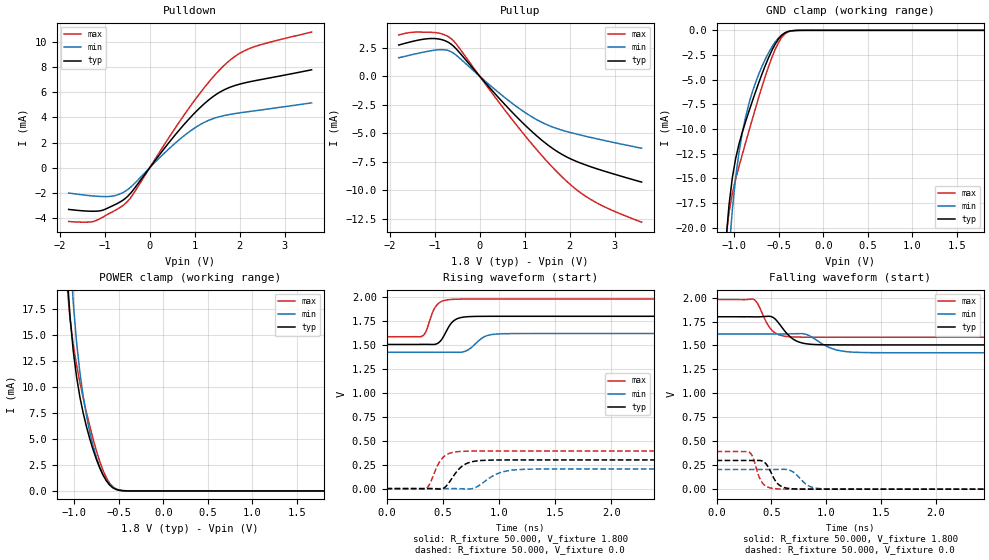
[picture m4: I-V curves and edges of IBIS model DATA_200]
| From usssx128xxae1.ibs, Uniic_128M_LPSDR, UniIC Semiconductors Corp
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|   Model DATA_200
[Model] DATA_200
Model_type I/O
Polarity   Inverting
Enable   Active-High
Vinl =  0.0V
Vinh =  1.800V
Vmeas =  0.900V
Vref =  0.900V
C_comp   1.060pF   1.050pF   1.070pF
[Model Spec]
Vinh   1.800V   1.400V   2.100V
Vinl   0.0V   -0.300V   0.400V
Vmeas   0.900V   0.810V   0.990V
Vref   0.900V   0.810V   0.990V
[Temperature Range]   25.000   0.125k   -40.000
[Voltage Range]   1.800V   1.620V   1.980V
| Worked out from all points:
|   slope of the pulldown table from 0 to 0.27 V, typ, clamps not added: 212 ohm
|   slope of the pullup table from 0 to 0.27 V, typ, clamps not added: 221 ohm
|   GND clamp passes 1 mA (typ) near -0.51 V on its own axis
|   POWER clamp passes 1 mA (typ) near -0.64 V on its own axis
|   rising waveform, R_fixture 50.000, V_fixture 1.800: 20-80 % time 91.8ps typ, 118ps min, 77.4ps max; typ from 1.51 V to 1.8 V
|   rising waveform, R_fixture 50.000, V_fixture 0.0: 20-80 % time 125ps typ, 171ps min, 97.4ps max; typ from 0 V to 0.3 V
|   falling waveform, R_fixture 50.000, V_fixture 1.800: 20-80 % time 139ps typ, 185ps min, 109ps max; typ from 1.8 V to 1.51 V
|   falling waveform, R_fixture 50.000, V_fixture 0.0: 20-80 % time 88.5ps typ, 114ps min, 72.7ps max; typ from 0.3 V to 0 V
[Pulldown]
|Voltage   I(typ)   I(min)   I(max)
-1.8V     -3.295mA   -1.994mA   -4.25mA
-1.195V   -3.435mA   -2.245mA   -4.185mA
-1.03V    -3.339mA   -2.275mA   -3.883mA
-810mV    -2.983mA   -2.23mA    -3.454mA
-480mV    -2.229mA   -1.703mA   -2.619mA
400mV     1.869mA    1.411mA    2.243mA
895mV     3.949mA    2.895mA    4.836mA
1.39V     5.592mA    3.872mA    7.11mA
1.83V     6.441mA    4.26mA     8.654mA
2.05V     6.676mA    4.38mA     9.168mA
2.325V    6.891mA    4.511mA    9.59mA
3.6V      7.767mA    5.147mA    10.75mA
[Pullup]
|Voltage   I(typ)   I(min)   I(max)
-1.8V     2.731mA    1.612mA    3.624mA
-1.46V    3.081mA    1.927mA    3.861mA
-1.075V   3.305mA    2.238mA    3.848mA
-855mV    3.219mA    2.33mA     3.728mA
-635mV    2.812mA    2.146mA    3.296mA
-470mV    2.17mA     1.67mA     2.561mA
905mV     -3.895mA   -2.906mA   -4.718mA
1.4V      -5.677mA   -4.087mA   -7.046mA
1.84V     -6.889mA   -4.75mA    -8.873mA
2.225V    -7.596mA   -5.151mA   -10.18mA
2.555V    -8.063mA   -5.453mA   -11.01mA
3.6V      -9.294mA   -6.325mA   -12.82mA
[GND_clamp]
|Voltage   I(typ)   I(min)   I(max)
-1.8V     -271.7mA   -304.3mA   -257.9mA
-1.097V   -21.71mA   -28.04mA   -21.32mA
-1.06V    -17.73mA   -22.52mA   -18.46mA
-1.023V   -14.97mA   -18.24mA   -16.55mA
-986mV    -13.03mA   -14.97mA   -15.09mA
-912mV    -10.37mA   -10.44mA   -12.62mA
-801mV    -7.262mA   -6.333mA   -9.099mA
-690mV    -4.437mA   -3.666mA   -5.721mA
-579mV    -2.043mA   -1.694mA   -2.765mA
-431mV    -248.4uA   -247.4uA   -345.1uA
-283mV    -5.293uA   -10.2uA    -5.65uA
1.8V      0A         0A         0A
[POWER_clamp]
|Voltage   I(typ)   I(min)   I(max)
-1.8V     340.2mA    394mA      317.1mA
-1.086V   21.52mA    29.62mA    20.16mA
-1.049V   16.79mA    23.07mA    16.54mA
-1.012V   13.42mA    18.08mA    14.02mA
-975mV    10.94mA    14.29mA    12.08mA
-938mV    9.034mA    11.39mA    10.43mA
-901mV    7.488mA    9.092mA    8.933mA
-827mV    5.01mA     5.66mA     6.217mA
-716mV    2.228mA    2.327mA    2.865mA
-568mV    301.3uA    355.6uA    397.2uA
-420mV    7.103uA    18.41uA    6.039uA
1.8V      0A         0A         0A
[Ramp]
| variable   typ   min   max
dV/dt_r   0.180/0.125n   0.123/0.171n   0.236/97.547p
dV/dt_f   0.176/0.139n   0.117/0.185n   0.236/0.110n
R_load = 50.000
[Rising Waveform]
R_fixture= 50.000
V_fixture= 1.800
V_fixture_min= 1.620
V_fixture_max= 1.980
|time   V(typ)   V(min)   V(max)
0s        1.506V     1.424V     1.586V
320ps     1.507V     1.424V     1.595V
353ps     1.507V     1.424V     1.647V
413ps     1.506V     1.424V     1.85V
443ps     1.511V     1.424V     1.912V
607ps     1.761V     1.424V     1.978V
713ps     1.795V     1.442V     1.98V
879ps     1.8V       1.592V     1.98V
1.031ns   1.8V       1.618V     1.98V
10ns      1.8V       1.62V      1.98V
[Rising Waveform]
R_fixture= 50.000
V_fixture= 0.0
V_fixture_min= 0.0
V_fixture_max= 0.0
|time   V(typ)   V(min)   V(max)
0s        16.25nV    102.8nV    27.47nV
352ps     578.9uV    32.05uV    -749.8uV
462ps     -4.438mV   4.627uV    259.9mV
502ps     991.9uV    179.1uV    325.3mV
580ps     104.6mV    506.8uV    375.5mV
706ps     259mV      -3.453mV   390.8mV
789ps     287.1mV    10.72mV    392.4mV
1.028ns   299.1mV    173.4mV    392.9mV
1.268ns   299.6mV    203.1mV    392.9mV
10ns      299.6mV    205.7mV    392.9mV
[Falling Waveform]
R_fixture= 50.000
V_fixture= 1.800
V_fixture_min= 1.620
V_fixture_max= 1.980
|time   V(typ)   V(min)   V(max)
0s        1.8V       1.62V      1.98V
337ps     1.799V     1.62V      1.982V
371ps     1.799V     1.62V      1.944V
462ps     1.804V     1.62V      1.726V
511ps     1.796V     1.62V      1.652V
701ps     1.564V     1.622V     1.589V
829ps     1.516V     1.611V     1.587V
1.087ns   1.506V     1.455V     1.586V
1.337ns   1.506V     1.426V     1.586V
10ns      1.506V     1.424V     1.586V
[Falling Waveform]
R_fixture= 50.000
V_fixture= 0.0
V_fixture_min= 0.0
V_fixture_max= 0.0
|time   V(typ)   V(min)   V(max)
0s        299.6mV    205.7mV    392.9mV
298ps     299.4mV    205.7mV    385.4mV
325ps     299.2mV    205.7mV    348.7mV
389ps     299.8mV    205.7mV    124.7mV
425ps     289.9mV    205.7mV    55.81mV
581ps     35.19mV    206.8mV    1.747mV
685ps     4.368mV    188.2mV    190.8uV
856ps     194.2uV    25.5mV     6.044uV
1.067ns   6.499uV    888.1uV    157.6nV
10ns      19.31nV    105.5nV    30.51nV
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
